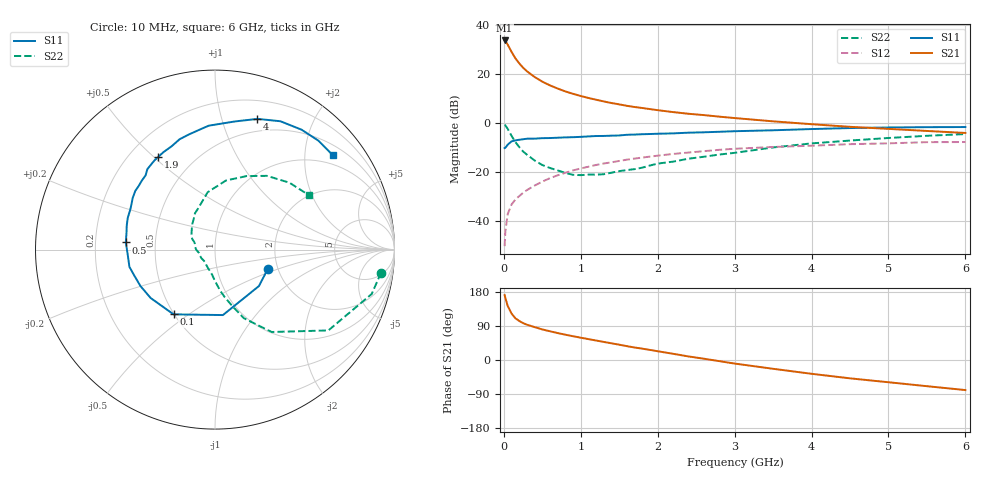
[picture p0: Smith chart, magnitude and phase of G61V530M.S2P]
! SIEMENS Small Signal Semiconductors
! BFG193
! Si NPN RF Bipolar Junction Transistor in SOT223
! VCE = 1.5 V  IC = 30 mA
! Common Emitter S-Parameters:  August  1996
# GHz  S  MA  R  50
!  f  S11  S21  S12  S22
! GHz  MAG  ANG  MAG  ANG  MAG  ANG  MAG  ANG
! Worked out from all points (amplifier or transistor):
!   36 points, 10 MHz to 6 GHz, reference 50 ohm
!   highest |S21| = 33.9 dB at 10 MHz (marker M1)
!   |S21| within 3 dB of that: start of sweep to 72.1 MHz
!   unconditionally stable (mu >= 1): 499.7 MHz to 2.692 GHz
!   at 250 MHz: K = 0.85, MSG = 25.6 dB, |S12| = -28.4 dB
!   at 1.4 GHz: K = 1.06, MAG = 10.6 dB, |S12| = -15.9 dB
!   at 6 GHz: K = 0.94, MSG = 1.9 dB, |S12| = -7.6 dB
!   S11 on the Smith chart (normalised r, x): 10 MHz: 1.77, -0.42; 100 MHz: 0.50, -0.44; 500 MHz: 0.34, +0.04; 1.9 GHz: 0.32, +0.52; 4 GHz: 0.37, +1.31; 6 GHz: 0.74, +2.67
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0.01  0.3132 -20.1  49.42 171.3  0.0031 89.0  0.934 -7.9
0.02  0.3181 -39.6  47.93 163.7  0.0062 78.8  0.9076 -15.8
0.05  0.3674 -83.1  40.61 142.8  0.014 69.0  0.7756 -35.5
0.1  0.4283 -122.6  28.98 122.7  0.022 61.0  0.557 -55.5
0.15  0.4487 -143.1  21.34 110.1  0.0278 59.0  0.4144 -67.2
0.2  0.4626 -154.1  16.84 103.0  0.0326 60.4  0.3288 -73.0
0.25  0.4735 -162.8  13.73 97.3  0.0381 60.7  0.2669 -78.8
0.3  0.4864 -168.6  11.62 93.2  0.0434 61.9  0.2299 -82.9
0.4  0.4875 -177.2  8.86 86.8  0.0536 62.5  0.1747 -90.1
0.5  0.4985 175.4  7.124 80.7  0.0646 62.7  0.141 -96.5
0.6  0.5015 169.6  5.97 75.8  0.0761 62.2  0.1226 -103.2
0.8  0.5172 160.1  4.495 66.8  0.0978 59.4  0.0974 -120.5
1.1  0.5414 147.9  3.303 55.1  0.1303 54.5  0.0898 -148.0
1.4  0.5609 136.4  2.603 44.1  0.1605 48.1  0.0984 -175.3
1.9  0.6062 121.3  1.957 26.6  0.2096 37.0  0.1378 155.7
2.2  0.6246 112.7  1.7 16.4  0.2374 29.7  0.1653 142.0
2.8  0.6735 97.4  1.373 -3.0  0.2882 15.4  0.2307 119.0
3.5  0.7224 81.2  1.101 -23.2  0.3296 -2.2  0.3222 97.3
4  0.7657 72.0  0.962 -36.4  0.3495 -11.9  0.3899 81.0
4.5  0.8026 63.0  0.85 -48.4  0.376 -21.9  0.4456 66.8
5.5  0.8368 46.5  0.7 -69.1  0.4131 -44.5  0.5574 42.0
6  0.8413 38.6  0.637 -79.4  0.4157 -57.5  0.6049 30.1
